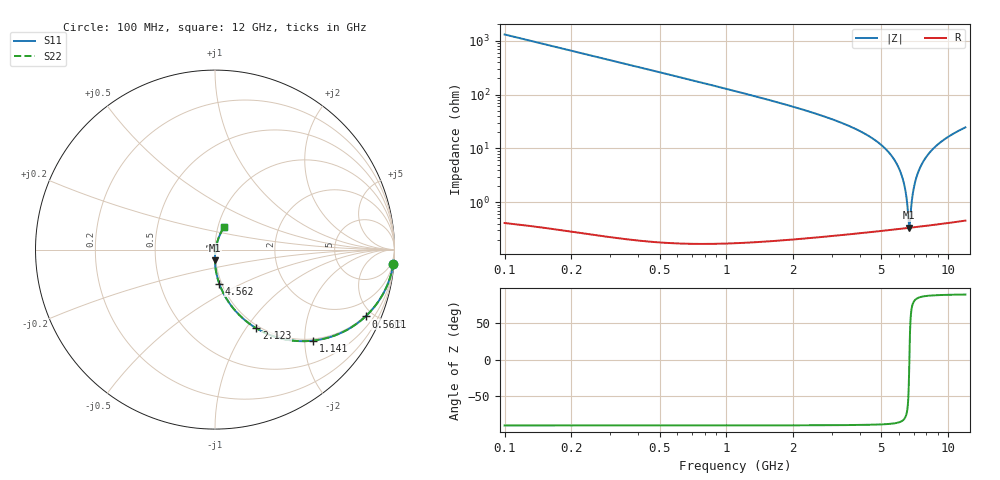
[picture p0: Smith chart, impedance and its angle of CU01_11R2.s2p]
! S-parameter model data by Modelithics Inc. support@modelithics.com 813-866-6335 Tampa FL USA
! S-Parameter data specifications:
! Substrate: 20-mil Rogers, substrate thickness, H=0.508mm, Dielectric constant, Er=3.75
! PCB Mounting Pad Footprint: Pad width, PadW=0.35mm , Pad length, PadL=0.30mm , Pad gap, PadG (edge-to-edge)=0.25mm , Reference planes=0.85mm apart
! Created Tue May  8 14:01:25 2018
# hz S ma R 50
! 2 Port Network Data from SP1.SP block
! freq  magS11  angS11  magS21  angS21  magS12  angS12  magS22  angS22
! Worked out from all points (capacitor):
!   801 points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, 100 MHz to 12 GHz, reference 50 ohm
!   read as one part in series: C = 1.22 pF near 159.5 MHz
!   lowest |Z| = 335 mohm at 6.705 GHz (marker M1)
!   series resonance near 6.705 GHz, so ESL is about 460 pH
!   S11 on the Smith chart (normalised r, x): 100 MHz: 1, -25; 561.1 MHz: 0.96, -4.52; 1.141 GHz: 0.96, -2.19; 2.123 GHz: 0.96, -1.12; 4.562 GHz: 0.97, -0.38; 12 GHz: 1.07, +0.28
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1e8  0.997 -4.5  0.07647 85.5  0.07647 85.5  0.997 -4.5
2.93375e8  0.9755 -13.0  0.2197 77.0  0.2197 77.0  0.9755 -13.0
5.61125e8  0.9177 -23.9  0.3966 66.0  0.3966 66.0  0.9177 -23.9
1.14125e9  0.7455 -42.9  0.6653 47.0  0.6653 47.0  0.7455 -42.9
1.602375e9  0.6155 -53.5  0.7866 36.4  0.7866 36.4  0.6155 -53.5
2.09325e9  0.5021 -61.8  0.863 28.0  0.863 28.0  0.5021 -61.8
2.123e9  0.496 -62.2  0.8665 27.6  0.8665 27.6  0.496 -62.2
2.956e9  0.3567 -71.8  0.932 17.9  0.932 17.9  0.3567 -71.8
4.071625e9  0.2323 -80.1  0.97 9.3  0.97 9.3  0.2323 -80.1
4.5625e9  0.1909 -82.8  0.9788 6.3  0.9788 6.3  0.1909 -82.8
6.05e9  0.09372 -88.9  0.9924 -0.8  0.9924 -0.8  0.09372 -88.9
6.7045e9  0.0596 -90.3  0.9948 -3.4  0.9948 -3.4  0.0596 -90.3
7.1805e9  0.03702 -89.9  0.9958 -5.2  0.9958 -5.2  0.03702 -89.9
7.5375e9  0.02115 -87.0  0.9962 -6.5  0.9962 -6.5  0.02115 -87.0
7.74575e9  0.01238 -80.6  0.9963 -7.2  0.9963 -7.2  0.01238 -80.6
7.98375e9  0.004044 -35.5  0.9963 -8.0  0.9963 -8.0  0.004044 -35.5
8.04325e9  0.003649 1.1  0.9963 -8.2  0.9963 -8.2  0.003649 1.1
8.34075e9  0.01315 64.6  0.9961 -9.2  0.9961 -9.2  0.01315 64.6
8.668e9  0.02572 71.3  0.9958 -10.3  0.9958 -10.3  0.02572 71.3
9.218375e9  0.04626 73.2  0.9949 -12.0  0.9949 -12.0  0.04626 73.2
1.002162e10  0.07469 72.4  0.993 -14.5  0.993 -14.5  0.07469 72.4
1.2e10  0.1387 68.0  0.9857 -20.2  0.9857 -20.2  0.1387 68.0
